|   IBIS model for TPS65930
[IBIS ver]   3.2
[File name]   tps65930.ibs
[File Rev]   0.2
[Date]   May 12,2009
[Source]   Data created at Texas Instruments
[Notes]   File originated from T2 ibis model and HSPICE simulation
   Oct 20,2008: First release
   May 12,2009: DP-DN model added Notes:
   -Some IV curves contain Non monotonic data points.
   They are appropriate spice simulation results.
   Extreme current warnings are not the problem. The currents
   correspond to the results of HSPICE simulation.
[Disclaimer]   This information is for modeling purpose only, and is not
   guaranteed. The information is subject to change without
   notice.
[Copyright]   Texas Instruments
|   Component TPS65930
[Component]   TPS65930
[Manufacturer]   Texas Instruments.
[Package]
|   variable   typ   min   max
R_pkg   9.14E-02   1.58E-01   2.02E-01
L_pkg   2.17E-09   1.12E-11   4.61E-09
C_pkg   1.15E-13   4.62E-13   1.85E-11
[Pin] signal_name 	model_name   R_pin	L_pin   C_pin
M10 32KCLKOUT		DIGIO_LOW_SPEED   8.280E-02  1.630E-09  8.470E-13
L14 32KXIN		NC   1.070E-01  2.210E-09  5.660E-13
K14 32KXOUT		NC   1.040E-01  2.330E-09  5.980E-13
H2  ADCIN0		NC   9.910E-02  1.990E-09  6.470E-13
F2  ADCIN2		NC   8.670E-02  1.630E-09  5.080E-13
K13 AGND		NC   8.860E-02  1.680E-09  9.750E-13
G1  AUXR		NC   9.390E-02  1.960E-09  5.050E-13
G2  AVSS1		NC   3.850E-02  1.090E-10  8.110E-12
L7  AVSS2		NC   2.490E-02  1.120E-11  7.130E-12
N14 AVSS3		NC   9.250E-02  2.820E-09  2.160E-12
C7  AVSS4		NC   2.020E-02  6.710E-10  1.580E-12
H9  BKBAT		NC   1.100E-01  2.860E-09  1.060E-12
E8  BOOT0		DIGIN50_VBAT   1.440E-01  4.290E-09  1.330E-12
D7  BOOT1		DIGIN50_VBAT   1.520E-01  4.060E-09  1.260E-12
E10 CLK256FS		DIGOUT_60MHZ   8.240E-02  1.710E-09  9.390E-13
A4  CLKEN		DIGOUT50   9.750E-02  2.380E-09  6.120E-13
B13 CLKREQ		DIGIN50_VIO_PPD   1.070E-01  2.650E-09  7.060E-13
N6  CPCAPM		NC   1.090E-01  2.090E-09  6.160E-13
N7  CPCAPP		NC   1.170E-01  2.590E-09  6.410E-13
P5  CPGND		NC   1.010E-01  2.170E-09  5.900E-13
P7  CPIN		NC   1.030E-01  2.220E-09  5.370E-13
L10 DATA0		DIGIO_50OHMS   1.190E-01  2.850E-09  9.190E-13
K10 DATA1		DIGIO_50OHMS   1.130E-01  2.460E-09  9.000E-13
G11 DATA2		DIGIO_50OHMS   1.130E-01  2.690E-09  9.660E-13
G10 DATA3		DIGIO_50OHMS   1.090E-01  2.630E-09  9.210E-13
E12 DATA4		DIGIO_50OHMS   1.160E-01  2.470E-09  9.460E-13
G9  DATA5		DIGIO_50OHMS   1.090E-01  2.620E-09  9.860E-13
G12 DATA6		DIGIO_50OHMS   1.130E-01  2.660E-09  9.700E-13
E11 DATA7		DIGIO_50OHMS   1.120E-01  2.770E-09  9.690E-13
H10 DGND		NC   3.260E-02  6.090E-11  1.850E-11
H11 DIR 		DIGOUT_50OHMS   9.950E-02  1.890E-09  7.380E-13
P10 DN_UART3TXD 	DN   1.580E-01  1.780E-09  5.300E-13
N10 DP_UART3RXD 	DP   1.550E-01  1.460E-09  6.610E-13
F7  GPIO0		DIGIO50_PPU_PPD   1.360E-01  4.310E-09  1.400E-12
E7  GPIO1		DIGIO50_PPU_PPD   1.530E-01  4.610E-09  1.510E-12
P13 GPIO15		DIGIO30_PPU_PPD   1.020E-01  2.960E-09  7.290E-13
P2  GPIO2		DIGIO30_PPU_PPD   1.300E-01  3.850E-09  7.720E-13
L5  GPIO6		DIGIO30_33M_PPU_PPD 8.060E-02  1.830E-09  9.940E-13
J7  GPIO7		DIGIO30_33M_PPU_PPD 1.400E-01  3.900E-09  1.250E-12
A11 HFCLKIN		NC   9.370E-02  2.070E-09  4.620E-13
M11 HFCLKOUT		DIGOUT50_50OHMS_HD  1.020E-01  2.170E-09  9.160E-13
B4  I2CCNTLSCL  	DIGIO50_SDA   7.880E-02  1.550E-09  7.580E-13
C3  I2CCNTLSDA  	DIGIO50_SDA   8.580E-02  1.790E-09  7.580E-13
H3  I2SCLK		DIGIO_LOW_SPEED   8.820E-02  1.570E-09  7.390E-13
K4  I2SDIN		DIGIN50_VIO   9.490E-02  2.030E-09  8.340E-13
K3  I2SDOUT		DIGOUT50   8.070E-02  1.690E-09  7.490E-13
K2  I2SSYNC		DIGIO50_STRONG   9.620E-02  1.850E-09  8.260E-13
G6  ID   NC   1.090E-01  3.610E-09  1.350E-12
C10 INT1		DIGOUT50   7.520E-02  1.260E-09  5.930E-13
B7  IO1P8		NC   5.420E-02  1.380E-09  2.120E-12
B14 JTAGTCK_BERCLK	DIGIN50_VIO   9.960E-02  2.070E-09  6.170E-13
A13 JTAGTDI_BERDATA	DIGIN50_VIO   7.700E-02  2.760E-09  2.730E-12
G4  KPDC0		DIGOUT_OD_PPU_3P1   1.050E-01  3.240E-09  1.080E-12
G3  KPDC1		DIGOUT_OD_PPU_3P1   8.450E-02  1.980E-09  9.510E-13
E5  KPDC2		DIGOUT_OD_PPU_3P1   8.770E-02  2.040E-09  9.120E-13
B2  KPDC3		DIGOUT_OD_PPU_3P1   8.620E-02  1.880E-09  8.510E-13
E3  KPDC4		DIGOUT_OD_PPU_3P1   7.650E-02  1.400E-09  7.580E-13
D5  KPDC5		DIGOUT_OD_PPU_3P1   1.030E-01  2.910E-09  9.980E-13
K7  KPDR0		DIGIN50_VIO_PPU   1.010E-01  2.540E-09  9.650E-13
H5  KPDR1		DIGIN50_VIO_PPU   1.150E-01  3.520E-09  1.220E-12
K5  KPDR2		DIGIN50_VIO_PPU   9.490E-02  2.220E-09  9.360E-13
H6  KPDR3		DIGIN50_VIO_PPU   1.080E-01  3.100E-09  1.180E-12
K8  KPDR4		DIGIN50_VIO_PPU   1.090E-01  2.380E-09  9.430E-13
L8  KPDR5		DIGIN50_VIO_PPU   1.160E-01  3.120E-09  1.240E-12
E13 LEDA_VIBRAP 	NC   7.740E-02  1.390E-09  6.430E-13
G13 LEDB_VIBRAM 	NC   7.840E-02  1.470E-09  6.790E-13
F13 LEDGND		NC   8.030E-02  1.530E-09  5.770E-13
B10 GPIO13_LEDSYNC	DIGIO30_33M_PPU_PPD 9.520E-02  2.500E-09  1.030E-12
E1  MICMAINM		NC   1.080E-01  2.440E-09  5.540E-13
D1  MICMAINP		NC   1.080E-01  2.600E-09  6.240E-13
D2  MICBIASGND  	NC   8.270E-02  1.750E-09  6.550E-13
E2  MICBIAS1OUT 	NC   7.430E-02  1.430E-09  4.960E-13
H4  MSECURE_VREF_AGND	DIGIN50_VIO   1.070E-01  3.470E-09  1.270E-12
C8  NRESPWRON		DIGOUT50   9.720E-02  2.030E-09  8.410E-13
B9  NRESWARM		DIGIN50_VIO   8.760E-02  1.770E-09  7.090E-13
G5  NSLEEP1		DIGIN50_VIO   1.340E-01  3.640E-09  1.190E-12
J8  NXT 		DIGOUT_50OHMS   1.170E-01  3.380E-09  1.140E-12
M5  PCHGAC		NC   8.060E-02  1.440E-09  6.900E-13
A7  PreDrivLEFT_VMID	NC   7.940E-02  1.720E-09  4.710E-13
A8  PreDrivRIGHT_ADCIN7 NC   9.700E-02  2.320E-09  5.690E-13
B3  PWROK2_I2CSRSDA	DIGIO50_OR_SDA   7.840E-02  1.580E-09  7.040E-13
D10 PWRON		DIGIN50_VBAT   7.940E-02  1.630E-09  7.480E-13
B8  REGEN		DIGOUT50_OD_BAT   9.790E-02  1.960E-09  5.410E-13
H12 STP 		DIGIO_50OHMS   8.060E-02  1.380E-09  6.800E-13
D8  SYSEN		DIGOUT_OD_PPU_3P1   8.390E-02  2.040E-09  9.320E-13
A1  TEST		DIGIN50_VIO_PPD   1.110E-01  2.640E-09  7.060E-13
P14 TESTRESET		DIGIN50_VBAT   1.060E-01  2.530E-09  6.490E-13
P1  TESTV1		NC   1.100E-01  2.910E-09  6.540E-13
A14 TESTV2		NC   9.360E-02  2.160E-09  7.020E-13
K11 UCLK		DIGOUT_50OHMS   9.480E-02  1.950E-09  8.170E-13
L1  VAUX12SIN		NC   6.520E-02  2.580E-09  7.600E-13
N2  VAUX2OUT		NC   1.240E-01  3.370E-09  7.600E-13
N5  VBAT		NC   7.900E-02  1.520E-09  5.500E-13
A10 VBATRIGHTLEFT	NC   2.260E-02  8.060E-10  1.410E-12
N9  VBATUSB		NC   7.710E-02  2.420E-09  1.190E-12
P8  VBUS		NC   8.860E-02  2.120E-09  5.240E-13
K1  VDACIN		NC   7.020E-02  2.710E-09  7.840E-13
L2  VDACOUT		NC   1.140E-01  2.670E-09  6.760E-13
A12 VDD1GND		NC   2.740E-02  1.520E-09  1.680E-12
D12 VDD1IN		NC   2.470E-02  1.400E-09  1.350E-12
C11 VDD1L		NC   2.890E-02  1.390E-09  1.740E-12
E14 VDD1OUT		NC   9.040E-02  1.980E-09  4.910E-13
N12 VDD2GND		NC   2.610E-02  1.480E-09  9.000E-13
M13 VDD2IN		NC   3.270E-02  1.430E-09  1.130E-12
N11 VDD2L		NC   3.130E-02  1.410E-09  8.150E-13
N13 VDD2OUT		NC   9.030E-02  1.890E-09  6.260E-13
H13 VINTIN		NC   1.350E-01  2.820E-09  6.690E-13
H1  VINTANA1OUT 	NC   1.230E-01  2.730E-09  6.490E-13
A5  VINTANA2OUT 	NC   5.590E-02  1.260E-09  2.010E-12
J13 VINTDIGOUT  	NC   1.330E-01  2.620E-09  6.300E-13
M7  VINTUSB1P5OUT	NC   1.110E-01  1.870E-09  6.020E-13
N8  VINTUSB1P8OUT	NC   1.200E-01  2.340E-09  6.240E-13
P3  VIOGND		NC   2.440E-02  1.390E-09  9.380E-13
M3  VIOIN		NC   3.370E-02  1.460E-09  1.120E-12
N4  VIOL		NC   3.620E-02  1.650E-09  8.300E-13
M4  VIOOUT		NC   7.890E-02  1.530E-09  8.140E-13
A2  VMMC1IN		NC   3.600E-02  9.950E-10  1.460E-12
B1  VMMC1OUT		NC   1.030E-01  2.520E-09  6.620E-13
E4  VMODE1		DIGIN50_VIO   8.190E-02  1.880E-09  9.900E-13
C5  VMODE2_I2CSR_SCL	DIGIO50_OR_SDA   7.530E-02  1.260E-09  6.400E-13
H14 VPLLA3RIN		NC   7.100E-02  2.260E-09  8.180E-13
G14 VPPL1OUT		NC   8.910E-02  1.920E-09  5.210E-13
N1  VPRECH		NC   4.660E-02  1.520E-09  1.610E-12
L13 VREF		NC   8.410E-02  1.490E-09  6.620E-13
K12 VRTCOUT		NC   1.350E-01  2.850E-09  9.460E-13
M8  VUSB3P1		NC   1.390E-01  3.310E-09  7.870E-13
[Model Selector] DIGIO_LOW_S_PPU_PPD
DIGIO_LOW_S_PPU   pullup disable and low speed mode
DIGIO_LOW_S_PPD   pullup disable and high speed mode
DIGIO_LOW_SPEED   pullup enabled and low speed mode
[Model Selector] DIGIO50_SDA
DIGIO_SDA_NPU_NHP   pullup disable and low speed mode
DIGIO_SDA_NPU_HP   pullup disable and high speed mode
DIGIO_SDA_PU_NHP   pullup enabled and low speed mode
   | input mode with pullup emulation when driving a"1"
DIGIO_SDA_PU_HP   pullup enabled and high speed mode
   | input mode with pullup emulation when driving a"1"
[Model Selector] DIGIO50_OR_SDA
DIGIO_SDA_NPU_NHP   pullup disable and low speed mode
DIGIO_SDA_NPU_HP   pullup disable and high speed mode
DIGIO_SDA_PU_NHP   pullup enabled and low speed mode
   | input mode with pullup emulation when driving a"1"
DIGIO_SDA_PU_HP   pullup enabled and high speed mode
   | input mode with pullup emulation when driving a"1"
DIGIO50   PWROK2 digital input
[Model Selector] DIGIN50_VIO_OR_SDA
DIGIO_SDA_NPU_NHP pullup disable and low speed mode
DIGIO_SDA_NPU_HP  pullup disable and high speed mode
DIGIO_SDA_PU_NHP   pullup enabled and low speed mode
   | input mode with pullup emulation when driving a"1"
DIGIO_SDA_PU_HP   pullup enabled and high speed mode
   | input mode with pullup emulation when driving a"1"
DIGIN50_VIO   VMODE2 digital input
[Model Selector]   DIGOUT_OD_PPU_3P1
DIGOUT_OD_PPU_3P1PU   Model with PU_EN_LOWV = 1
DIGOUT_OD_PPU_3P1PUZ   Model with PU_EN_LOWV = 0
[Model Selector]   DIGOUT_60MHZ
DIGOUT_60MHZ_LDRIVE   Model with HDRIVE_LOWV=0 (drive 10pF load)
DIGOUT_60MHZ_HDRIVE   Model with HDRIVE_LOWV=1 (drive 30pF load)
[Model Selector]  DIGOUT50_OD_BAT
DIGOUT50_OD_BAT0  PU_EN_LOWV=1
DIGOUT50_OD_BAT1  PU_EN_LOWV=0
[Model Selector]  DIGIO_OD_PPU_3P1
DIGIO_OD_PPU_3P1PU  cell  PMOS_EN_LOWV=1  PU_EN_LOWV=1
DIGIO_OD_PPU_3P1PD  cell  PMOS_EN_LOWV=1  PU_EN_LOWV=0
DIGIO_OD_PPU_3P1OP  cell  PMOS_EN_LOWV=0  PU_EN_LOWV=1
[Model Selector]  DIGIO50_PPU_PPD_10
DIGIO50_PPU_PPD_10_0   Cell with PU_EN_LOWV=0, PD_EN_LOWV=0
DIGIO50_PPU_PPD_10_1   Cell with PU_EN_LOWV=1, PD_EN_LOWV=0
DIGIO50_PPU_PPD_10_2   Cell with PU_EN_LOWV=0, PD_EN_LOWV=1
[Model Selector]   DIGIN50_VBAT
DIGIN50_VBAT0   cell  with pu_en_lowv=0
DIGIN50_VBAT1   cell  with pu_en_lowv=1
[Model Selector]  DIGIO30_33M_PPU_PPD
DIGIO30_33M_PPU_PPD0   Cell with PU_EN_LOWV=0, PD_EN_LOWV=0
DIGIO30_33M_PPU_PPD1   Cell with PU_EN_LOWV=1, PD_EN_LOWV=0
DIGIO30_33M_PPU_PPD2   Cell with PU_EN_LOWV=0, PD_EN_LOWV=1
[Model Selector]   DIGIO30_PPU_PPD
DIGIO30_PPU_PPD_00   cell  with pu=0 and pd=0
DIGIO30_PPU_PPD_01   cell  with pu=0 and pd=1
DIGIO30_PPU_PPD_10   cell  with pu=1 and pd=0
[Model Selector]  DIGIO50_PPU_PPD
DIGIO50_PPU_PPD0   Cell with PU_EN_LOWV=0, PD_EN_LOWV=0
DIGIO50_PPU_PPD1   Cell with PU_EN_LOWV=1, PD_EN_LOWV=0
DIGIO50_PPU_PPD2   Cell with PU_EN_LOWV=0, PD_EN_LOWV=1
[Model Selector] DIGOUT50_50OHMS_HD
DIGOUT50_50OHMS_HD_L   Cell operated with pin HDRIVE_LOWV = LOW
DIGOUT50_50OHMS_HD_H   Cell operated with pin HDRIVE_LOWV = HIGH
[Model Selector] DP
DP_LS   Cell operated in Low Speed mode
DP_FS   Cell operated in Full Speed mode
DP_HS   Cell operated in High Speed mode
[Model Selector] DN
DN_LS   Cell operated in Low Speed mode
DN_FS   Cell operated in Full Speed mode
DN_HS   Cell operated in High Speed mode
| Models and submodels in the file (48): DIGIO_SDA_NPU_NHP (I/O_open_drain), DIGIO_SDA_NPU_HP (I/O_open_drain), DIGIO_SDA_PU_HP (Output), DIGIO_SDA_PU_NHP (Output), DIGOUT50_50OHMS_HD_L (3-state), DIGOUT50_50OHMS_HD_H (3-state), DIGIO_LOW_SPEED (I/O), DIGIO_LOW_S_PPU (I/O), DIGIO_LOW_S_PPD (I/O), DIGIO_50OHMS (I/O), DIGOUT_50OHMS (3-state), DIGOUT_OD_PPU_3P1PU (I/O_open_drain), DIGOUT_OD_PPU_3P1PUZ (I/O_open_drain), DIGOUT_60MHZ_LDRIVE (3-state), DIGOUT_60MHZ_HDRIVE (3-state), DIGOUT50_OD_BAT0 (3-state), DIGOUT50_OD_BAT1 (3-state), DIGIO_OD_PPU_3P1PU (I/O), DIGIO_OD_PPU_3P1PD (I/O), DIGIO_OD_PPU_3P1OP (I/O), DIGIO50_STRONG (I/O), DIGIO50_PPU_PPD_10_0 (I/O), DIGIO50_PPU_PPD_10_1 (I/O), DIGIO50_PPU_PPD_10_2 (I/O), DIGIO50_PPU_PPD0 (I/O), DIGIO50_PPU_PPD1 (I/O), DIGIO50_PPU_PPD2 (I/O), DIGIO50 (I/O), DIGIO30_PPU_PPD_00 (I/O), DIGIO30_PPU_PPD_01 (I/O), DIGIO30_PPU_PPD_10 (I/O), DIGIO30_33M_PPU_PPD0 (I/O), DIGIO30_33M_PPU_PPD1 (I/O), DIGIO30_33M_PPU_PPD2 (I/O), DIGIN50_VIO_PPU (Input), DIGIN50_VIO_PPD (Input), DIGIN50_VIO (Input), DIGIN50_VBAT0 (Input), DIGIN50_VBAT1 (Input), DIGIN50_3P1 (Input), DIGIN50 (Input), DIGOUT50 (3-state), DP_LS (3-state), DN_LS (3-state), DP_FS (3-state), DN_FS (3-state), DP_HS (I/O_open_source), DN_HS (I/O_open_source)
